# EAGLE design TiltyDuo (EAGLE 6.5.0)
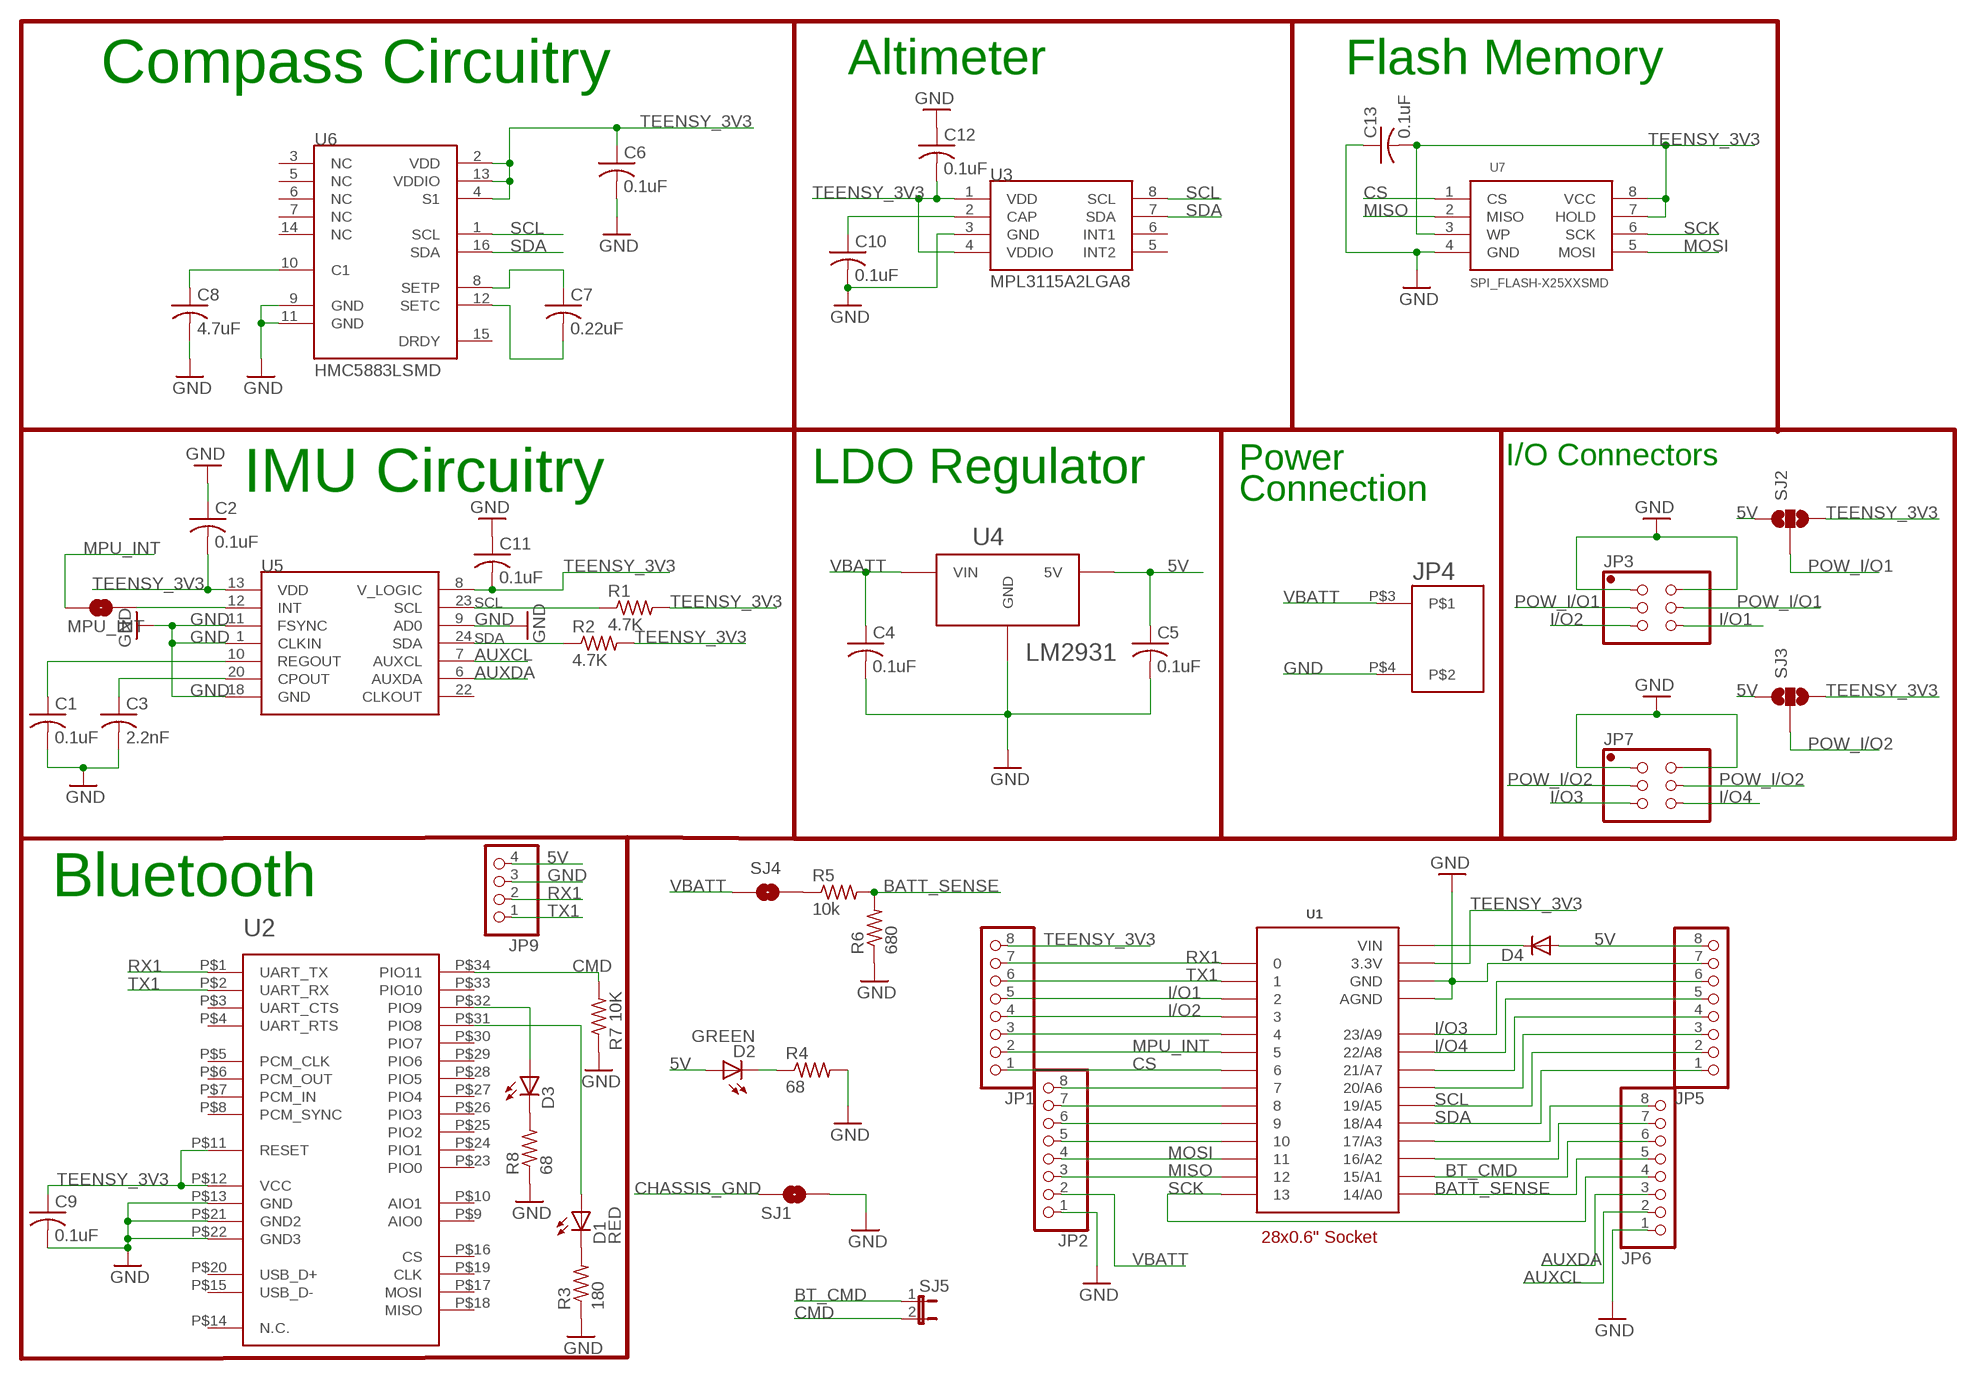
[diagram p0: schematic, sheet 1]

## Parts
C1  0.1uF  C-USC0603  [C0603]
C2  0.1uF  C-USC0603  [C0603]
C3  2.2nF  C-USC0603  [C0603]
C4  0.1uF  C-USC0603  [C0603]
C5  0.1uF  C-USC0603  [C0603]
C6  0.1uF  C-USC0603  [C0603]
C7  0.22uF  C-USC0603  [C0603]
C8  4.7uF  C-USC0603  [C0603]
C9  0.1uF  C-USC0603  [C0603]
C10  0.1uF  C-USC0603  [C0603]
C11  0.1uF  C-USC0603  [C0603]
C12  0.1uF  C-USC0603  [C0603]
C13  0.1uF  C-USC0603  [C0603]
D1  RED  LED-GREENLED-0805_NO_SILK  [LED-0805]
D2  GREEN  LED-GREENLED-0805_NO_SILK  [LED-0805]
D3  YELLOW  LED-GREENLED-0805_NO_SILK  [LED-0805]
D4  DIODESOT23  [SOT23-3]
JP1  PINHD-1X81X08_NO_SILK_LOCK  [1X08_NO_SS_LOCKING]
JP2  PINHD-1X81X08_NO_SILK_LOCK  [1X08_NO_SS_LOCKING]
JP3  PINHD-2X32X03_NO_SS_LOCK  [2X03_NO_SS_LOCK]
JP4  2-POS_SMD_TERM_BLOCK  [2-POS_SMD_TERMINAL_BLOCK]
JP5  PINHD-1X81X08_NO_SILK_LOCK  [1X08_NO_SS_LOCKING]
JP6  PINHD-1X81X08_NO_SILK_LOCK  [1X08_NO_SS_LOCKING]
JP7  PINHD-2X32X03_NO_SS_LOCK  [2X03_NO_SS_LOCK]
JP9  PINHD-1X41X04_NO_SS_LOCKING  [1X04_NO_SS_LOCKING]
MPU_INT  SOLDERJUMPERNO  [SJ_2S-NO]
R1  4.7K  R-US_R0603  [R0603]
R2  4.7K  R-US_R0603  [R0603]
R3  180  R-US_R0603  [R0603]
R4  68  R-US_R0603  [R0603]
R5  10k  R-US_R0603  [R0603]
R6  680  R-US_R0603  [R0603]
R7  10K  R-US_R0603  [R0603]
R8  68  R-US_R0603  [R0603]
SJ1  SOLDERJUMPERNO  [SJ_2S-NO]
SJ2  SOLDERJUMPER_2WAYS  [SJ_3]
SJ3  SOLDERJUMPER_2WAYS  [SJ_3]
SJ4  SOLDERJUMPERTRACE  [SJ_2S-TRACE]
SJ5  JUMPER-2SMD-NC  [SJ_2S]
U1  TEENSY_3.0_OUTER-PINS28-DIP_SOCKET  [28-DIP]
U2  HC-09_BREAKOUT  [HC-09_BREAKOUT]
U3  MPL3115A2LGA8  [LGA8]
U4  LM2931  [TO263]
U5  MPU-6050  [QFN-24]
U6  HMC5883LSMD  [16LPCC]
U7  SPI_FLASH-X25XXSMD  [SO08]

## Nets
5V: C5.1 D2.1(A) D4.1(A) JP5.8 JP9.4 SJ2.1 SJ3.1 U4.P$3(5V)
AUXCL [I/O]: JP6.2 U5.7(AUXCL)
AUXDA [I/O]: JP6.3 U5.6(AUXDA)
BATT_SENSE: JP6.5 R5.2 R6.2 U1.P$27(14/A0)
BT_CMD: JP6.6 SJ5.1 U1.P$26(15/A1)
CHASSIS_GND: SJ1.1
CMD: R7.2 SJ5.2 U2.P$34(PIO11)
CS: JP1.1 U1.P$8 U7.1(CS)
GND: C1.2 C2.1 C3.2 C4.2 C5.2 C6.2 C8.2 C9.2 C10.2 C11.1 C12.1 C13.1 JP2.1 JP3.1 JP3.2 JP4.P$4 JP5.7 JP6.1 JP7.1 JP7.2 JP9.3 R3.1 R4.2 R6.1 R7.1 R8.1 SJ1.2 U1.P$1(GND) U1.P$16(AGND) U2.P$13(GND) U2.P$21(GND2) U2.P$22(GND3) U3.3(GND) U4.P$1(GND) U5.1(CLKIN) U5.9(AD0) U5.11(FSYNC) U5.18(GND) U6.9(GND) U6.11(GND) U7.4(GND)
I/O1: JP1.5 JP3.6 U1.P$4
I/O2: JP1.4 JP3.5 U1.P$5
I/O3: JP5.6 JP7.5 U1.P$18(23/A9)
I/O4: JP5.5 JP7.6 U1.P$19(22/A8)
MISO: JP2.3 U1.P$14 U7.2(MISO)
MOSI: JP2.4 U1.P$13 U7.5(MOSI)
MPU_INT: JP1.2 MPU_INT.1 U1.P$7
N$1: C1.1 U5.10(REGOUT)
N$2: C3.1 U5.20(CPOUT)
N$3: D1.2(C) R3.2
N$5: C7.1 U6.8(SETP)
N$6: C7.2 U6.12(SETC)
N$7: JP1.3 U1.P$6
N$8: JP2.5 U1.P$12
N$9: R5.1 SJ4.2
N$10: JP6.8 U1.P$24(17/A3)
N$11: C8.1 U6.10(C1)
N$12: JP2.6 U1.P$11
N$13: D2.2(C) R4.1
N$14: D1.1(A) U2.P$31(PIO8)
N$15: D4.3(C) U1.P$15(VIN)
N$16: MPU_INT.2 U5.12(INT)
N$18: JP5.4 U1.P$20(21/A7)
N$19: JP5.3 U1.P$21(20/A6)
N$21: C10.1 U3.2(CAP)
N$23: JP6.7 U1.P$25(16/A2)
N$24: D3.2(C) R8.2
POW_I/O1: JP3.3 JP3.4 SJ2.2
POW_I/O2: JP7.3 JP7.4 SJ3.2
RX1: JP1.7 JP9.2 U1.P$2 U2.P$1(UART_TX)
RX3: JP2.8 U1.P$9
SCK: JP6.4 U1.P$28 U7.6(SCK)
SCL [I/O]: JP5.2 R1.1 U1.P$22(19/A5) U3.8(SCL) U5.23(SCL) U6.1(SCL)
SDA [I/O]: JP5.1 R2.1 U1.P$23(18/A4) U3.7(SDA) U5.24(SDA) U6.16(SDA)
TEENSY_3V3 [3.3V]: C2.2 C6.1 C9.1 C11.2 C12.2 C13.2 JP1.8 R1.2 R2.2 SJ2.3 SJ3.3 U1.P$17(3.3V) U2.P$11(RESET) U2.P$12(VCC) U3.1(VDD) U3.4(VDDIO) U5.8(V_LOGIC) U5.13(VDD) U6.2(VDD) U6.4(S1) U6.13(VDDIO) U7.3(WP) U7.7(HOLD) U7.8(VCC)
TX1: JP1.6 JP9.1 U1.P$3 U2.P$2(UART_RX)
TX3: JP2.7 U1.P$10
VBATT: C4.1 JP2.2 JP4.P$3 SJ4.1 U4.P$2(VIN)
YEL_LED: D3.1(A) U2.P$32(PIO9)
Unconnected: U2.P$3(UART_CTS) U2.P$4(UART_RTS) U2.P$5(PCM_CLK) U2.P$6(PCM_OUT) U2.P$7(PCM_IN) U2.P$8(PCM_SYNC) U2.P$9(AIO0) U2.P$10(AIO1) U2.P$14(N.C.) U2.P$15(USB_D-) U2.P$16(CS) U2.P$17(MOSI) U2.P$18(MISO) U2.P$19(CLK) U2.P$20(USB_D+) U2.P$23(PIO0) U2.P$24(PIO1) U2.P$25(PIO2) U2.P$26(PIO3) U2.P$27(PIO4) U2.P$28(PIO5) U2.P$29(PIO6) U2.P$30(PIO7) U2.P$33(PIO10) U3.5(INT2) U3.6(INT1) U5.22(CLKOUT) U6.3(NC) U6.5(NC) U6.6(NC) U6.7(NC) U6.14(NC) U6.15(DRDY)

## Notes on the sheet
- Compass Circuitry | Altimeter | Flash Memory
- Power | I/O Connectors
- IMU Circuitry | LDO Regulator
- Connection
- Bluetooth
- 28x0.6" Socket

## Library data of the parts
C1 C6 C9 C10 C13 = resistor:C-US: CAPACITOR, American symbol; RATED_VOLTAGE: 2
C2 C4 C5 C11 C12 = resistor:C-US: CAPACITOR, American symbol
C3 = resistor:C-US: CAPACITOR, American symbol; RATED_VOLTAGE: 50
C7 C8 = resistor:C-US: CAPACITOR, American symbol; ESR: <200mOhms
D1-D3 = SparkFun-LED:LED-GREEN: Various green LEDs
D4 = SparkFun-DiscreteSemi:DIODE: Diode
JP1 JP2 JP5 JP6 = pinhead:PINHD-1X8: PIN HEADER
JP3 JP7 = pinhead:PINHD-2X3: PIN HEADER
JP4 = My Parts:2-POS_SMD_TERM_BLOCK; PART#: 277-2337-1-ND; POSSIBLE_ALT: 009276002021106
JP9 = pinhead:PINHD-1X4: PIN HEADER
MPU_INT SJ1 SJ4 = SparkFun-Passives:SOLDERJUMPER: Solder Jumper
R1-R8 = resistor:R-US_: RESISTOR, American symbol
SJ2 SJ3 = SparkFun-Passives:SOLDERJUMPER_2WAY: Solder Jumper 2 way solder jumper
SJ5 = SparkFun-Passives:JUMPER-2: Jumper
U1 = My Parts:TEENSY_3.0_OUTER-PINS; COST: 0.28; PART#: AE10004-ND; PART#2: A28-LC-TR-R; PART#3: ED3052-5-ND
U2 = csr:HC-09_BREAKOUT
U3 = SparkFun-Sensors:MPL3115A2: Altimeter/Pressure Sensor, I2C, 1.95V-3.6V supply, 50 to 110kPa
U4 = on-semiconductor:LM2931; COST: 0.53
U5 = SparkFun-Sensors:MPU-6050: MPU-6000 - I2C address is 0x68 with AD0 low and 0x69 with AD0 high.
U6 = SparkFun:HMC5883L: 3 Axis Digital Compass IC
U7 = SparkFun-DigitalIC:SPI_FLASH-X25XX: 8pin SPI Flash series x25xx. Works with devices like W25X32 and BR25L32; PART#: S25FL204K0TMFI043

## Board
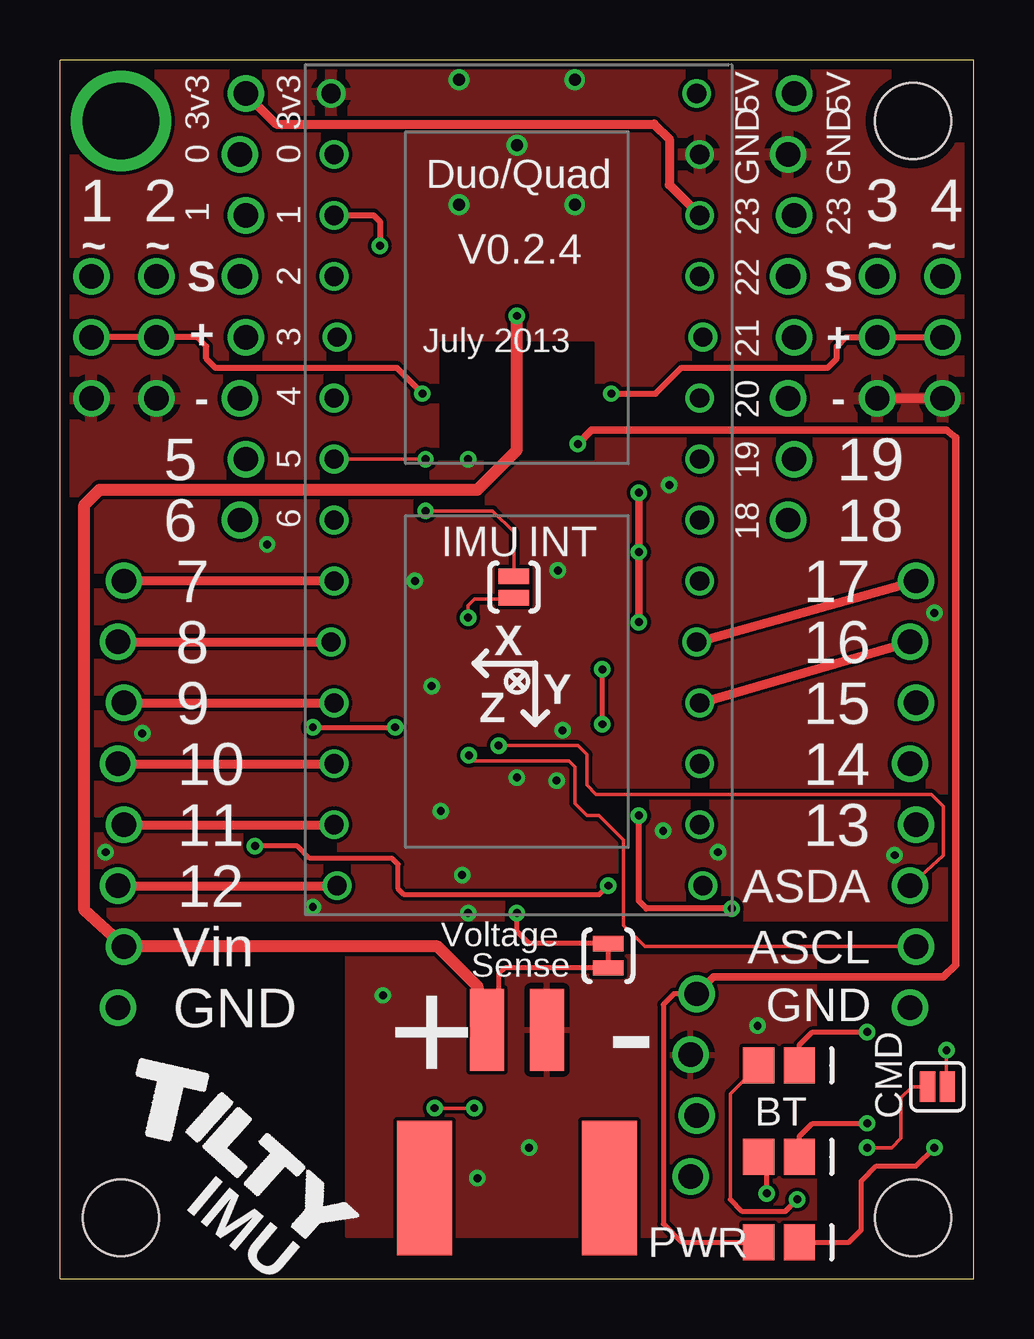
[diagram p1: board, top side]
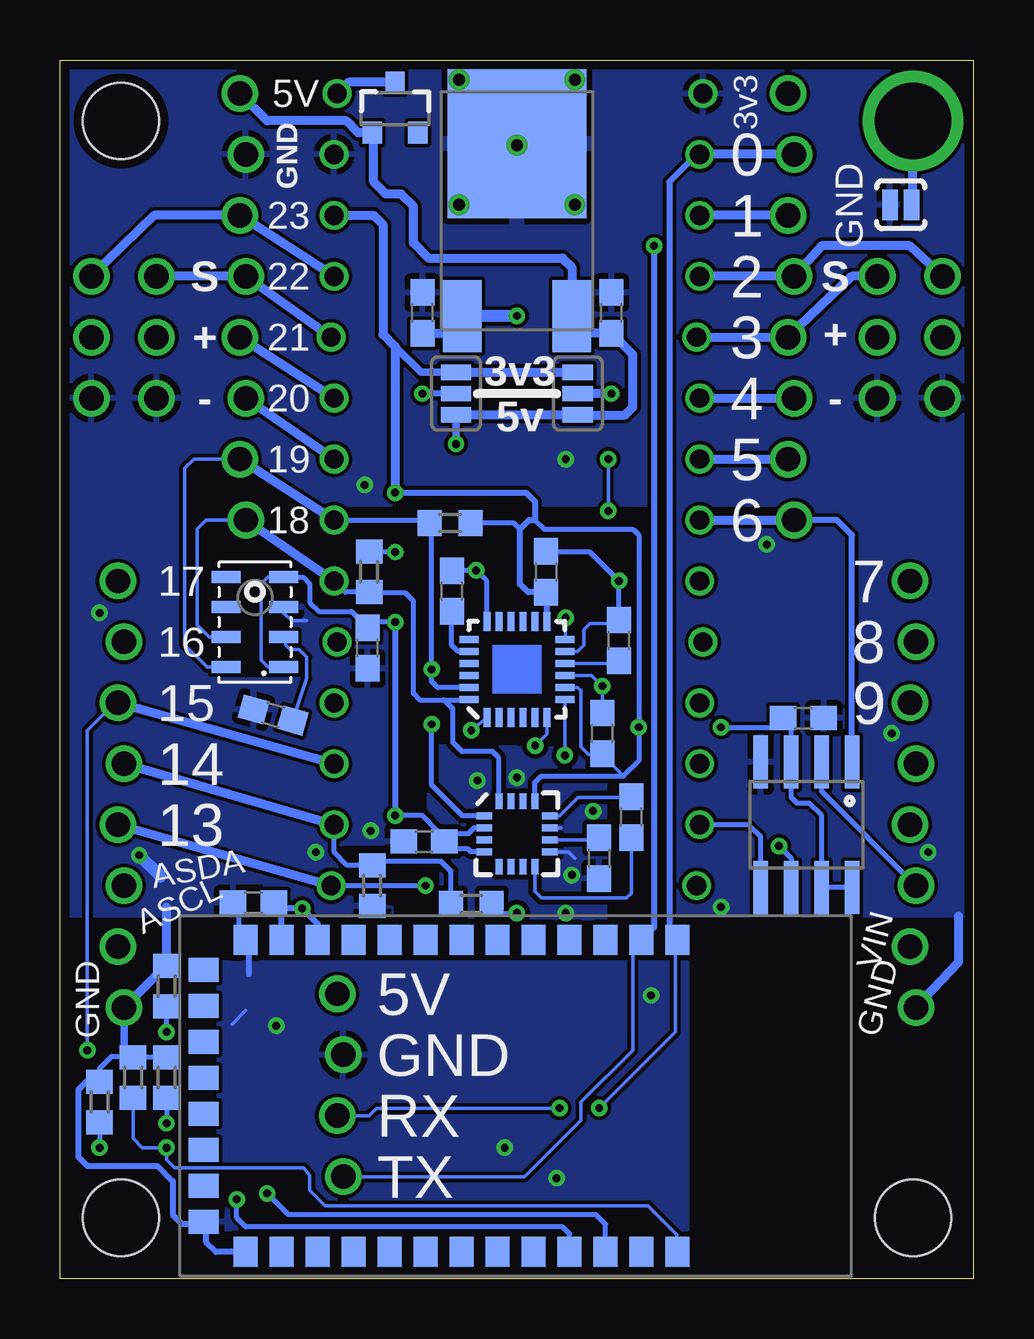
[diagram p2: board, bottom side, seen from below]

Size 38.1 x 50.8 mm. Coordinates in mm from the lower left corner, seen from the top.
Outline: 0,0 38.1,0 38.1,50.8 0,50.8 0,0
Copper layers (1*16): Top 0.0356mm / dielectric 1.5011mm / Bottom 0.0356mm
Design rules "LaenPCBOrder": minimum track width 6mil, minimum drill 13mil, track to track 6mil, track to pad 6mil, pad to pad 6mil, via to via 6mil, smd to smd 6mil, copper to edge 15mil, drill to drill 6mil, minimum pad ring 7mil, minimum via ring 7mil, stop-mask expansion 4mil, vias tented up to drill 0mil, thermal gap 10mil
Holes 3.17 mm at 35.56,48.26 35.56,2.54 2.54,2.54

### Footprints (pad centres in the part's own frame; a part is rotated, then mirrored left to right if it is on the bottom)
C0603 = smd 1.1 x 1: 1 -0.85,0; 2 0.85,0
LED-0805 = smd 1.3 x 1.5: 1 -0.85,0; 2 0.85,0
SOT23-3 = smd 0.8 x 0.9: 1 -0.95,-1; 2 0.95,-1; 3 0,1.1
1X08_NO_SS_LOCKING = drill 1.016: 1 -8.89,0.127; 2 -6.35,-0.127; 3 -3.81,0.127; 4 -1.27,-0.127; 5 1.27,0.127; 6 3.81,-0.127; 7 6.35,0.127; 8 8.89,-0.127
2X03_NO_SS_LOCK = drill 1.016: 1 -2.54,-1.359; 2 -2.54,1.359; 3 0,-1.359; 4 0,1.359; 5 2.54,-1.359; 6 2.54,1.359
2-POS_SMD_TERMINAL_BLOCK = smd 2.3 x 5.6: P$1 -3.85,-2.325; P$2 3.85,-2.325 | smd 1.4 x 3.4: P$3 -1.25,4.275; P$4 1.25,4.275
1X04_NO_SS_LOCKING = drill 1.016: 1 -3.81,0.127; 2 -1.27,-0.127; 3 1.27,0.127; 4 3.81,-0.127
SJ_2S-NO = smd 0.635 x 1.27: 1 -0.45,0; 2 0.45,0
R0603 = smd 1 x 1.1: 1 -0.85,0; 2 0.85,0
SJ_3 = smd 0.635 x 1.27: 1 -0.889,0; 2 0,0; 3 0.889,0
SJ_2S-TRACE = smd 0.635 x 1.27: 1 -0.508,0; 2 0.508,0
SJ_2S = smd 0.635 x 1.27: 1 -0.412,0; 2 0.412,0
28-DIP = drill 0.8: P$1 -7.747,16.51; P$2 -7.62,13.97; P$3 -7.62,11.43; P$4 -7.62,8.89; P$5 -7.493,6.35; P$6 -7.62,3.81; P$7 -7.62,1.27; P$8 -7.62,-1.27; P$9 -7.62,-3.81; P$10 -7.747,-6.35; P$11 -7.62,-8.89; P$12 -7.62,-11.43; P$13 -7.62,-13.97; P$14 -7.493,-16.51; P$15 7.493,16.51; P$16 7.62,13.97; P$17 7.62,11.43; P$18 7.62,8.89; P$19 7.747,6.35; P$20 7.62,3.81; P$21 7.62,1.27; P$22 7.62,-1.27; P$23 7.62,-3.81; P$24 7.493,-6.35; P$25 7.62,-8.89; P$26 7.62,-11.43; P$27 7.62,-13.97; P$28 7.747,-16.51
HC-09_BREAKOUT = smd 1.25 x 1: P$1 -6.5,10.5; P$2 -6.5,9; P$3 -6.5,7.5; P$4 -6.5,6; P$5 -6.5,3; P$6 -6.5,4.5; P$7 -6.5,1.5; P$8 -6.5,0; P$9 -6.5,-1.5; P$10 -6.5,-3; P$11 -6.5,-4.5; P$12 -6.5,-6; P$13 -6.5,-7.5; P$22 6.5,-7.5; P$23 6.5,-6; P$24 6.5,-4.5; P$25 6.5,-3; P$26 6.5,-1.5; P$27 6.5,0; P$28 6.5,1.5; P$29 6.5,3; P$30 6.5,4.5; P$31 6.5,6; P$32 6.5,7.5; P$33 6.5,9; P$34 6.5,10.5 | smd 1 x 1.25: P$14 -5.25,-9.25; P$15 -3.75,-9.25; P$16 -2.25,-9.25; P$17 -0.75,-9.25; P$18 0.75,-9.25; P$19 2.25,-9.25; P$20 3.75,-9.25; P$21 5.25,-9.25
LGA8 = smd 1.2 x 0.5: 1 -1.2,1.875; 2 -1.2,0.625; 3 -1.2,-0.625; 4 -1.2,-1.875; 5 1.2,-1.875; 6 1.2,-0.625; 7 1.2,0.625; 8 1.2,1.875
TO263 = smd 5.791 x 6.198: P$1 0,2.794 | smd 1.6 x 2.997: P$2 -2.286,-4.394; P$3 2.286,-4.394
QFN-24 = smd 0.8 x 0.3: 1 -2,1.25; 2 -2,0.75; 3 -2,0.25; 4 -2,-0.25; 5 -2,-0.75; 6 -2,-1.25; 13 2,-1.25; 14 2,-0.75; 15 2,-0.25; 16 2,0.25; 17 2,0.75; 18 2,1.25 | smd 0.3 x 0.8: 7 -1.25,-2; 8 -0.75,-2; 9 -0.25,-2; 10 0.25,-2; 11 0.75,-2; 12 1.25,-2; 19 1.25,2; 20 0.75,2; 21 0.25,2; 22 -0.25,2; 23 -0.75,2; 24 -1.25,2
16LPCC = smd 0.65 x 0.28: 1 -1.37,0.75; 2 -1.37,0.25; 3 -1.37,-0.25; 4 -1.37,-0.75; 9 1.37,-0.75; 10 1.37,-0.25; 11 1.37,0.25; 12 1.37,0.75 | smd 0.28 x 0.65: 5 -0.75,-1.37; 6 -0.25,-1.37; 7 0.25,-1.37; 8 0.75,-1.37; 13 0.75,1.37; 14 0.25,1.37; 15 -0.25,1.37; 16 -0.75,1.37
SO08 = smd 0.61 x 2.21: 1 -1.905,-2.616; 2 -0.635,-2.616; 3 0.635,-2.616; 4 1.905,-2.616; 5 1.905,2.616; 6 0.635,2.616; 7 -0.635,2.616; 8 -1.905,2.616

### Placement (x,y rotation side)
C1  14.8,26.61 90 bottom
C2  17.84,29.46 270 bottom
C3  21.75,28.66 90 bottom
C4  22.99,40.26 90 bottom
C5  15.11,40.26 90 bottom
C6  22.92,18.22 180 bottom
C7  14.29,19.24 90 bottom
C8  15.62,17.53 270 bottom
C9  30.04,15.68 180 bottom
C10  29.21,23.5 164.1 bottom
C11  15.49,22.73 270 bottom
C12  25.27,26.29 90 bottom
C13  7.11,23.37 180 bottom
D1  29.97,8.89 0 top
D2  29.97,1.52 0 top
D3  29.97,5.08 0 top
D4  24.13,48.77 0 bottom
JP1  7.62,40.51 90 top
JP2  2.54,20.19 90 top
JP3  2.67,39.24 90 top
JP4  19.05,6.1 0 top
JP5  30.48,40.51 90 top
JP6  35.56,20.19 90 top
JP7  35.43,39.24 90 top
JP9  26.42,8.06 90 top
MPU_INT  18.92,28.83 270 top
R1  21.84,31.5 0 bottom
R2  25.21,29.46 90 bottom
R3  33.66,12.19 270 bottom
R4  36.45,7.37 90 bottom
R5  20.95,15.62 180 bottom
R6  25.08,16.38 90 bottom
R7  35.05,8.38 270 bottom
R8  33.66,8.38 270 bottom
SJ1  3.05,44.77 180 bottom
SJ2  16.51,36.89 90 bottom
SJ3  21.59,36.89 90 bottom
SJ4  22.86,13.46 90 top
SJ5  36.58,8 180 top
U1  19.05,32.89 0 top
U2  22.86,7.62 270 bottom
U3  29.97,27.37 180 bottom
U4  19.05,44.51 0 bottom
U5  19.05,25.4 90 bottom
U6  19.05,18.54 0 bottom
U7  6.99,18.92 180 bottom

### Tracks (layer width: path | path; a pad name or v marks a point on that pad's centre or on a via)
5V  (via drill 0.33)
  Top 0.203: D2.1 25.91,1.52 25.15,2.29 25.15,11.43 25.59,11.87 JP9.4
  Top 0.305: 36.83,12.57 37.34,13.08
  Top 0.318: 37.34,13.08 37.34,35.05 36.96,35.37 22.16,35.37 v21.59,34.8 | 36.83,12.57 27.24,12.57 JP9.4
  Bottom 0.318: SJ3.1 v21.59,34.8
  Bottom 0.381: SJ3.1 SJ2.1 14.54,36.01 14.22,36.32 14.22,38.52 C5.1 16.76,39.41 U4.P$3 16.76,42.16 17.14,42.55 22.73,42.55 23.37,43.18 23.37,44.7 23.88,45.21 24.51,45.21 25.02,45.72 25.02,47.71 D4.1 25.67,47.77 26.16,48.26 29.46,48.26 JP5.8
  Bottom 0.508: 16.75,40.17 U4.P$3 16.71,40.17
AUXCL  (via drill 0.33)
  Top 0.152: v17.05,21.81 17.27,21.59 21.21,21.59 21.46,21.34 21.46,19.81 21.97,19.3 22.48,19.3 23.5,18.29 23.5,14.73 24.38,13.84 JP6.2
  Bottom 0.152: U5.7 v17.05,21.81
AUXDA  (via drill 0.33)
  Top 0.152: JP6.3 36.83,17.65 36.83,19.68 36.32,20.19 22.35,20.19 21.97,20.57 21.97,21.84 21.59,22.23 v18.29,22.23
  Bottom 0.152: 17.78,23.38 U5.6 17.8,22.71 v18.29,22.23
BATT_SENSE
  Bottom 0.203: 24.99,17.46 R6.2 | R6.2 26.12,17.23 26.67,17.78 U1.P$27 | R5.2 21.8,16.98 22.23,17.4 25.04,17.4 R6.2
  Bottom 0.381: U1.P$27 JP6.5
BT_CMD  (via drill 0.33)
  Top 0.152: v36.96,9.53 36.96,8.03 SJ5.1
  Bottom 0.152: JP6.6 35.81,24 36.96,22.86 v36.96,9.53
  Bottom 0.381: U1.P$26 JP6.6
CHASSIS_GND  (via drill 3.17)
  Bottom 0.381: SJ1.1 2.6,44.96 2.54,45.02 v2.54,48.26
CMD  (via drill 0.33)
  Top 0.152: v33.66,5.46 34.67,5.46 35.05,5.84 R7.2 35.52,8 SJ5.2
  Bottom 0.152: U2.P$34 12.38,1.1 12.38,1.84 13.59,3.05 27.05,3.05 27.69,3.68 27.69,4.32 27.94,4.62 33.33,4.62 33.66,4.95 v33.66,5.46 34.67,5.46 35.05,5.84 R7.2 | 12.38,1.14 U2.P$34 | 12,0.64 U2.P$34
CS
  Bottom 0.203: 5,21.46 U7.1
  Bottom 0.254: U7.1 5.08,30.99 5.71,31.62 JP1.1
  Bottom 0.381: U1.P$8 JP1.1
GND  (via drill 0.33, 0.51 pad 0.18)
  Top 0.381: JP7.2 JP7.1
  Bottom 0.152: U5.9 15.94,25.15 v15.49,24.7 C11.1 | 30.92,10.6 30.35,11.18 | U6.9 16.9,17.79 16.64,17.53 | U5.11 16.52,26.15 16.26,26.42 16.26,27.05 16,27.3 15.07,27.3 C1.2 | U3.3 28.77,27.76 28.45,27.43 27.81,27.43 | U6.11 17.47,18.79 17.21,18.8 | 20.32,23.38 v20.95,22.86
  Bottom 0.203: U2.P$13 30.63,14.39 30.63,15.43 C9.2 | C2.1 17.82,30.29 16,30.29 v14.8,29.08 C1.2 | U5.18 20.3,29.08 v20.75,29.53 21.74,29.53 C3.2 | R8.1 R7.1 35.09,9.27 35.94,9.27 36.45,8.76 R4.2
  Bottom 0.254: 20.32,23.38 U5.1 | U2.P$22 31.6,1.12 32,1.52 32,2.26 U2.P$21 32.19,2.29 33.02,2.29 33.4,2.67 33.4,4.06 34.04,4.7 36.96,4.7 37.34,5.08 37.34,7.87 37,8.22 R4.2 | U2.P$13 | U2.P$13 30.36,13.98 | U2.P$13 30.23,14.11 30.23,12.7 | 30.57,14.33 U2.P$13 | 15.47,16.7 C8.2
  Bottom 0.318: JP6.1 35.43,9.61 R7.1
  Bottom 0.381: JP2.1 0.64,13.21 0.64,15.11 | JP6.1 33.72,13.02 R3.1 33.66,15.49
  Bottom 0.508: 33.91,16.76 v34.8,17.65
  other vias: 19.05,47.24 16.64,44.77 21.46,44.77 21.46,49.97 16.64,49.97 15.88,19.49 17.4,4.19 13.46,11.81 16.76,16.83 25.15,18.67 25.4,33.08 8.64,30.61 17.02,34.16 27.43,17.78 19.56,5.46 1.91,17.78 3.43,22.73 29.08,10.54 17.02,15.24 10.54,15.49 20.7,20.76 19.05,20.89 36.45,27.75
  pour Top (isolate 0.127): 0,50.8 38.1,50.8 38.1,15.11 0,15.11
  pour Bottom: 0,32.26 0,50.8 38.1,50.8 38.1,32.26
  pour Bottom: 0,32.26 13.59,32.26 13.59,15.11 0,15.11
  pour Bottom: 24.13,32.26 37.97,32.26 38.1,15.11 24.26,15.11
  pour Top: 11.94,13.46 31.5,13.46 31.5,1.78 11.94,1.78
  pour Bottom: 11.94,2.03 11.94,13.21 31.5,13.21 31.5,12.57 31.5,2.03
  pour Bottom (isolate 0.203): 15.37,22.1 22.73,22.23 22.73,15.11 15.37,14.99
  pour Bottom: 16,50.29 22.1,50.29 22.1,43.94 16,43.94
I/O1
  Bottom 0.381: U1.P$4 JP1.5 6.35,43.05 2.67,43.05 JP3.6
I/O2
  Bottom 0.381: U1.P$5 JP1.4 5.08,41.78 JP3.5
I/O3
  Bottom 0.381: U1.P$18 JP5.6 34.16,44.32 JP7.5
I/O4
  Bottom 0.381: U1.P$19 JP5.5 JP7.6
MISO
  Top 0.381: JP2.3 U1.P$14
  Bottom 0.203: JP2.3 6.35,20.32 U7.2
MOSI
  Top 0.381: JP2.4 U1.P$13
  Bottom 0.203: U7.5 8.89,18.41 9.4,18.92 U1.P$13
MPU_INT  (via drill 0.33)
  Top 0.152: MPU_INT.1 18.92,31.11 18.03,32 v15.24,32 | v15.24,34.16 U1.P$7
  Bottom 0.152: v15.24,32 v15.24,34.16
  Bottom 0.381: U1.P$7 JP1.2
N$1
  Bottom 0.152: U5.10 14.9,25.65 C1.1
N$2
  Bottom 0.203: U5.20 21.52,26.15 21.78,26.42 21.78,27.79 C3.1
N$3  (via drill 0.33)
  Top 0.203: D1.2 30.82,9.74 31.37,10.29 v33.66,10.29
  Bottom 0.203: v33.66,10.29 R3.2
N$4
  cutout Bottom: 17.53,20.07 17.53,17.02 20.57,17.02 20.57,20.07
N$5
  Bottom 0.152: C7.1 14.29,16.07 14.48,15.88 18.03,15.88 18.3,16.14 U6.8
N$6
  Bottom 0.152: U6.12 17.28,19.29 16.51,20.07 14.31,20.07 C7.2
N$7
  Bottom 0.381: U1.P$6 JP1.3
N$8
  Top 0.381: JP2.5 U1.P$12
N$9  (via drill 0.33)
  Top 0.203: SJ4.2 19.56,13.97 19.05,14.48 v19.05,15.24
  Bottom 0.152: v19.05,15.24 19.72,15.24 R5.1
N$10
  Top 0.381: U1.P$24 JP6.8
N$11
  Bottom 0.152: U6.10 15.2,18.29 C8.1
N$12
  Top 0.381: JP2.6 U1.P$11
N$13  (via drill 0.33)
  Top 0.203: D2.2 32.89,1.52 33.4,2.03 33.4,4.06 34.04,4.7 35.69,4.7 v36.45,5.46
  Bottom 0.203: R4.1 v36.45,5.46
N$14  (via drill 0.33)
  Top 0.152: 27.94,3.3 27.94,7.71 D1.1
  Top 0.203: v30.73,3.3 30.23,2.79 28.45,2.79 27.94,3.3
  Bottom 0.203: U2.P$31 16.86,1.87 17.14,2.16 30.35,2.16 30.73,2.54 v30.73,3.3
N$15
  Bottom 0.381: D4.3 26.08,49.87 U1.P$15
N$16  (via drill 0.33)
  Top 0.152: v17.02,27.56 17.02,28.07 17.27,28.32 18.86,28.32 MPU_INT.2
  Bottom 0.152: v17.02,27.56 17.02,26.68 U5.12
N$18
  Bottom 0.381: U1.P$20 JP5.4
N$19
  Bottom 0.381: U1.P$21 JP5.3
N$20
  cutout Top: 15.88,38.99 22.23,38.99 22.23,34.16 15.88,34.16
N$21
  Bottom 0.152: 28.78,26.86 U3.2 28.7,26.8 28.7,26.42 28.51,26.23 28.13,26.23 27.81,25.91 27.81,25.02 C10.1
N$23
  Top 0.381: U1.P$25 JP6.7
N$24  (via drill 0.33)
  Top 0.203: D3.2 30.82,5.93 31.37,6.48 v33.66,6.48
  Bottom 0.203: R8.2 v33.66,6.48
N$25
  cutout Bottom: 29.72,15.24 29.72,16.38 30.35,16.38 30.35,15.24
N$26
  cutout Bottom: 22.35,15.11 26.29,16.13 26.29,17.97 22.35,17.97
N$28
  cutout Bottom: 28.57,29.84 31.37,29.84 31.37,25.15 28.57,25.15
POW_I/O1  (via drill 0.33)
  Top 0.254: JP3.4 JP3.3 5.71,39.24 6.1,38.86 6.1,38.35 6.48,37.97 14.03,37.97 v15.11,36.89
  Bottom 0.381: v15.11,36.89 SJ2.2
POW_I/O2  (via drill 0.33)
  Top 0.254: JP7.3 JP7.4 32.77,39.24 32.38,38.86 32.38,38.35 32,37.97 25.91,37.97 24.83,36.89 v22.99,36.89
  Bottom 0.254: SJ3.2 v22.99,36.89
RX1  (via drill 0.33)
  Top 0.152: v17.27,7.11 v15.62,7.11
  Bottom 0.152: 12.38,14.1 U2.P$1 12.45,14.03 12.45,10.29 v15.62,7.11 | JP9.2 25.21,6.79 24.89,7.11 v17.27,7.11
  Bottom 0.254: U1.P$2 11.56,46.86 12.7,45.72 12.7,14.59 U2.P$1
  Bottom 0.381: JP1.7 U1.P$2
RX3
  Top 0.381: U1.P$9 JP2.8
SCK  (via drill 0.33)
  Top 0.203: v22.86,16.38 22.48,16 14.35,16 14.1,16.26 14.1,17.27 13.84,17.53 10.41,17.53 9.91,18.03 v8.13,18.03
  Bottom 0.203: v22.86,16.38 U1.P$28 | v8.13,18.03 7.62,17.53 U7.6
  Bottom 0.381: U1.P$28 JP6.4
SCL  (via drill 0.33)
  Top 0.203: 30.48,34.16 JP5.2 | v22.61,23.11 v22.61,25.4
  Bottom 0.152: JP5.2 32.51,34.16 32.89,33.78 32.89,26.42 31.97,25.49 U3.8
  Bottom 0.203: U5.23 21.06,24.64 22.35,24.64 22.61,24.89 v22.61,25.4 22.61,31.41 R1.1 22.82,31.62 U1.P$22 | U6.1 21.32,19.29 22.61,20.57 v22.61,23.11
  Bottom 0.381: U1.P$22 JP5.2
SDA
  Bottom 0.152: JP5.1 32,31.62 32.38,31.24 32.38,27.24 31.89,26.74 U3.7
  Bottom 0.203: 22.1,24.13 23.11,24.13 23.37,24.38 23.37,28.26 23.69,28.57 25.17,28.57 R2.1 26.2,28.61 U1.P$23 | 22.1,24.13 21.07,24.13 U5.24 | U6.16 19.8,21.7 20.07,21.97 21.34,21.97 21.72,22.35 21.72,23.75 22.1,24.13
  Bottom 0.381: U1.P$23 JP5.1
TEENSY_3V3  (via drill 0.33)
  Top 0.203: v10.54,22.99 v13.97,22.99
  Top 0.254: v28,15.43 24.45,15.43 24.13,15.75 v24.13,19.3
  Top 0.305: v24.13,32.77 v24.13,30.29 v24.13,27.37
  Top 0.381: JP1.8 9.02,48.13 24.77,48.13 25.4,47.5 25.4,45.59 U1.P$17
  Bottom 0.152: U5.8 16.52,24.65 16.38,24.51 16.38,22.16 16.07,21.84 15.53,21.84 | 15.53,21.84 C11.2 | 15.53,21.84 14.61,20.95 | U3.1 29.43,25.49 29.72,25.78 29.72,28.96 29.43,29.24 U3.4
  Bottom 0.203: U6.4 20.97,17.79 21.08,17.91 21.76,17.91 C6.1 | U6.2 20.83,18.79 21.08,18.54 21.76,18.54 C6.1 | 18.29,31.62 17.91,31.24 14.22,31.24 13.97,30.99 v13.97,22.99 13.97,21.59 14.61,20.95 18.03,20.95 18.3,20.69 U6.13 | C6.1 22.29,18.22 22.35,18.29 22.35,18.67 22.99,19.3 v24.13,19.3 | v24.13,27.37 25.04,27.37 C12.2 25.95,27.81 27.3,27.81 27.69,28.19 27.69,28.96 27.97,29.24 U3.4 28.74,29.34 | 18.92,31.24 19.18,31.5 R1.2 | v24.13,30.29 25.18,30.29 R2.2 | U7.8 U7.7 6.35,19.3 6.86,19.81 7.37,19.81 7.62,20.07 U7.3 7.62,23.37 C13.2 8.09,22.99 v10.54,22.99
  Bottom 0.254: U5.13 17.8,28.57 C2.2 18.58,28.61 18.92,28.96 18.92,31.24 18.54,31.62 18.29,31.62 18.29,32.38 18.67,32.77 v24.13,32.77 | U2.P$11 27.36,14.79 v28,15.43 28.93,15.43 C9.1 28.86,15.36 U2.P$12 | v24.13,27.37 v24.13,19.3
  Bottom 0.318: SJ3.3 23.05,37.78 24.13,38.86
  Bottom 0.381: v24.13,32.77 24.13,38.86 24.64,39.37 24.64,43.94 25.02,44.32 U1.P$17 | SJ3.3 SJ2.3
TX1  (via drill 0.33)
  Top 0.254: U1.P$3 13.08,44.32 13.34,44.07 v13.34,43.05
  Bottom 0.152: JP9.1 18.73,4.25 16.38,6.6 16.38,7.37 14.22,9.53 14.22,13.76 U2.P$2
  Bottom 0.254: v13.34,43.05 13.34,14.64 U2.P$2
  Bottom 0.381: JP1.6 U1.P$3
TX3
  Top 0.381: JP2.7 U1.P$10
VBATT  (via drill 0.33)
  Top 0.203: SJ4.1 18.54,12.95 18.29,12.7 18.29,10.86 JP4.P$3
  Top 0.508: JP4.P$3 17.4,10.77 17.4,12.19 15.75,13.84 JP2.2 1.02,15.37 1.02,32.26 1.65,32.89 17.4,32.89 19.05,34.54 v19.05,40.13
  Bottom 0.381: C4.1 21.34,39.41 U4.P$2
  Bottom 0.508: v19.05,40.13 21.29,40.13 U4.P$2 21.4,40.18
YEL_LED  (via drill 0.33)
  Top 0.203: v29.46,3.56 29.46,4.74 D3.1
  Bottom 0.203: U2.P$32 15.36,2.28 15.75,2.67 28.57,2.67 v29.46,3.56

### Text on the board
tNames: 5V | 5V | 3v3 | 3v3 | 0 | 0 | Duo/Quad | GND | GND | 1 | 2 | 3 | 4 | 1 | 1 | V0.2.4 | 23 | 23 | ~ | ~ | S | S | ~ | ~ | 2 | 22 | + | 3 | July 2013 | + | 21 | - | - | 4 | 20 | 5 | 5 | 19 | 19 | 6 | 18 | 6 | IMU | INT | 18 | 17 | 7 | 16 | 8 | X | Y | 15 | 9 | Z | 10 | 14 | 13 | 11 | ASDA | 12 | Vin | Voltage | ASCL | Sense | GND | GND | + | - | BT | CMD | IMU | PWR
bNames: 5V | 3v3 | GND | 0 | GND | 1 | 23 | S | 2 | 22 | S | + | 3 | 21 | + | 3v3 | - | 4 | 20 | - | 5v | 5 | 19 | 6 | 18 | 7 | 17 | 8 | 16 | 9 | 15 | 14 | 13 | ASDA | ASCL | VIN | 5V | GND | GND | GND | RX | TX

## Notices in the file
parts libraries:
SparkFun-Sensors: Licensing: CC v3.0 Share-Alike You are welcome to use this library for commercial purposes.
